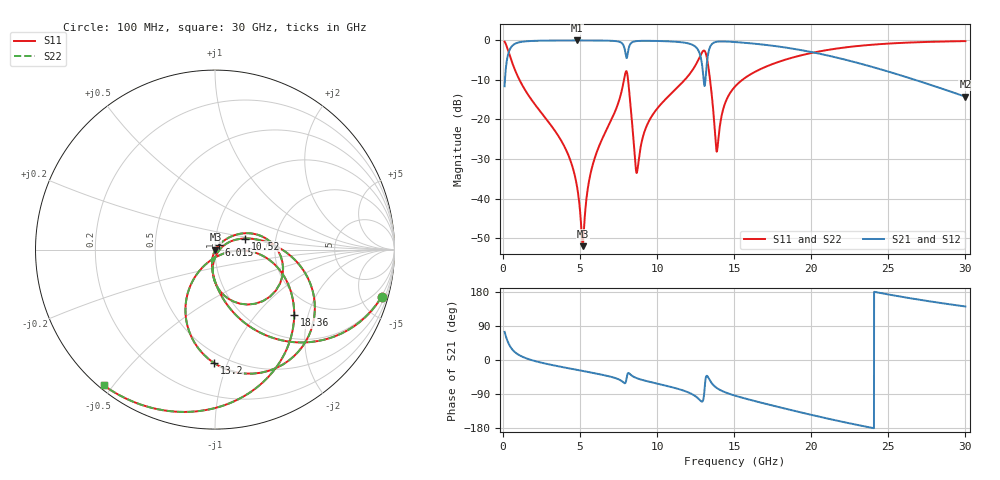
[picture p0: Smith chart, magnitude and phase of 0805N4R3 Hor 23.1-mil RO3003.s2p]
# GHz S MA R 50
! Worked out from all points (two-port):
!   3201 points, 100 MHz to 30 GHz, reference 50 ohm
!   highest |S21| = -0.02 dB at 4.819 GHz (marker M1); lowest = -14.2 dB at 30 GHz (marker M2)
!   |S21| within 3 dB of the highest: 364.4 MHz to 7.933 GHz (7.569 GHz wide, 182 % of centre); 13.33 GHz to 20.1 GHz (6.769 GHz wide, 40.5 % of centre)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
!   lowest |S11| = -52.0 dB at 5.164 GHz (marker M3), VSWR 1.01, Z = 50.2 - j0.127 ohm
!   |S11| at or under -10 dB: 1.066 GHz to 7.845 GHz (6.778 GHz wide, 152 % of centre); 8.111 GHz to 11.79 GHz (3.675 GHz wide, 36.9 % of centre); 13.43 GHz to 15.52 GHz (2.087 GHz wide, 14.4 % of centre)
!   |S22| runs from -52.0 to -0.2 dB; largest |S21 - S12| = 0
!   S11 on the Smith chart (normalised r, x): 100 MHz: 0.93, -7.07; 6.015 GHz: 1.05, +0.06; 10.52 GHz: 1.39, +0.18; 13.2 GHz: 0.43, -0.90; 18.36 GHz: 1.50, -1.64; 30 GHz: 0.01, -0.47
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0.1  0.9646 -15.8  0.2634 74.1  0.2634 74.1  0.9646 -15.8
0.5671875  0.5392 -60.5  0.8416 29.4  0.8416 29.4  0.5392 -60.5
1.099781  0.307 -78.2  0.9507 11.7  0.9507 11.7  0.307 -78.2
3.921594  0.04794 -106.9  0.9967 -19.3  0.9967 -19.3  0.04794 -106.9
4.818594  0.01347 -106.3  0.9974 -26.2  0.9974 -26.2  0.01347 -106.3
5.089563  0.003838 -78.4  0.9973 -28.3  0.9973 -28.3  0.003838 -78.4
5.164313  0.002505 -30.3  0.9973 -28.9  0.9973 -28.9  0.002505 -30.3
6.014594  0.0356 49.2  0.9959 -35.5  0.9959 -35.5  0.0356 49.2
7.64975  0.2108 25.6  0.9408 -54.2  0.9408 -54.2  0.2108 25.6
7.958094  0.3993 -18.5  0.6615 -58.9  0.6615 -58.9  0.3993 -18.5
8.677563  0.02114 -29.3  0.9796 -48.0  0.9796 -48.0  0.02114 -29.3
10.06978  0.1426 24.0  0.982 -63.0  0.982 -63.0  0.1426 24.0
10.51828  0.1783 20.3  0.976 -67.3  0.976 -67.3  0.1783 20.3
12.15344  0.386 -1.1  0.9 -87.8  0.9 -87.8  0.386 -1.1
12.78881  0.633 -28.6  0.6519 -106.5  0.6519 -106.5  0.633 -28.6
13.19994  0.6337 -90.3  0.459 -42.0  0.459 -42.0  0.6337 -90.3
13.87269  0.03934 -59.1  0.9615 -74.0  0.9615 -74.0  0.03934 -59.1
15.05  0.2605 -6.8  0.9525 -94.0  0.9525 -94.0  0.2605 -6.8
18.35769  0.5734 -39.7  0.8099 -128.8  0.8099 -128.8  0.5734 -39.7
20.03956  0.6948 -55.8  0.7097 -145.1  0.7097 -145.1  0.6948 -55.8
25.01978  0.911 -97.7  0.402 172.8  0.402 172.8  0.911 -97.7
30  0.9783 -129.3  0.1941 141.2  0.1941 141.2  0.9783 -129.3
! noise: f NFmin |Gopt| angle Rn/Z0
0.1  0.0008018  0.924  1.236  0.002338
3.417  0.005954  0.6891  19.52  0.00362
6.743  0.0139  0.7358  37.22  0.009467
10.06  0.02035  0.7386  54.34  0.01241
13.39  0.1179  0.9353  71.17  0.2688
16.7  0.02954  0.7236  85.01  0.01177
20.03  0.03515  0.7323  98.23  0.01158
23.35  0.04568  0.7677  111.1  0.01328
26.67  0.06237  0.8134  123.9  0.01602
30  0.09014  0.8624  136.7  0.01976
